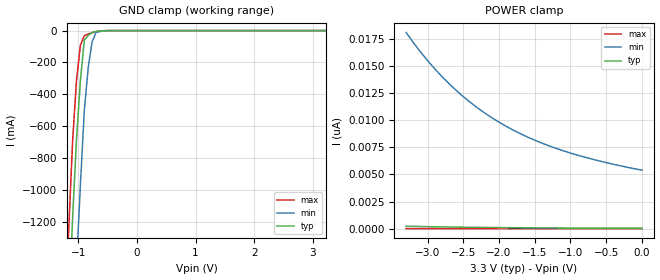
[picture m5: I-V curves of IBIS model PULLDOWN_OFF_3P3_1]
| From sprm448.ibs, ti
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|   Model Cell PULLDOWN_OFF_3P3
|PULLDOWN_OFF_3P3
[Model]   PULLDOWN_OFF_3P3_1
Model_type   Input
Polarity   Non-Inverting
Vinl =  0.8v
Vinh =  2v
C_comp   2.1697p   1.9812p   2.6822p
[Model Spec]
Vinl   0.8v   0.8v   0.8v
Vinh   2v   2v   2v
[Temperature Range]   25   125   -40
[Voltage Range]   3.3   3   3.6
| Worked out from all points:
|   GND clamp passes 1 mA (typ) near -0.56 V on its own axis
[POWER_clamp]
|   voltage   I(typ)   I(min)   I(max)
-3.3V     227.6pA    18.1nA     4.698pA
-3.2V     212.5pA    17.18nA    4.414pA
-3V       185.5pA    15.5nA     3.766pA
-2.7V     151.7pA    13.37nA    2.771pA
-2.4V     125.3pA    11.64nA    2.256pA
-2.2V     110.4pA    10.66nA    2.052pA
-2V       98.04pA    9.819nA    1.661pA
-1.8V     87.33pA    9.085nA    1.377pA
-1.6V     78.06pA    8.446nA    1.208pA
-1.2V     63.5pA     7.402nA    1.075pA
-700mV    50.45pA    6.416nA    737.2fA
-11.55fV  37.67pA    5.389nA    461.9fA
[GND_clamp]
|   voltage   I(typ)   I(min)   I(max)
-3.3V     -22.4A     -23.17A    -21.98A
-1.233V   -2.327A    -3.192A    -1.823A
-1.167V   -1.741A    -2.598A    -1.245A
-1.1V     -1.17A     -2.014A    -689.7mA
-1.033V   -680.3mA   -1.468A    -310.2mA
-966.7mV  -310.2mA   -963.5mA   -90.83mA
-900mV    -59.62mA   -500.1mA   -31.74mA
-833.3mV  -29.87mA   -231.2mA   -21.87mA
-766.7mV  -12.05mA   -68.61mA   -13.38mA
-700mV    -6.168mA   -12.26mA   -6.287mA
-433.3mV  -64.49uA   -229.1uA   -21.15uA
3.233V    36.77pA    5.7nA      404.1fA
